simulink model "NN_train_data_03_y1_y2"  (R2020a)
settings: Solver=VariableStepAuto  StartTime=0.0  StopTime=300  RelTol=1e-3
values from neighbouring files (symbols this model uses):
  C = 6.3000e-04    (= 0.00063)    [maglev_init.m]
  g = 9.80    (= 9.8)    [maglev_init.m]
  K = 1.0e+03 * [-2.4567   -0.1235    0.0237]    [maglev_init.m]
  L1 = 0.6000    (= 0.6)    [maglev_init.m]
  m = 0.0300    (= 0.03)    [maglev_init.m]
  mpert = 0    [maglev_init.m]
  R = 45    [maglev_init.m]
  Ts = 0.005    [maglev_init.m]    (also in train_net.m)
  x1_0 = 0.1    [maglev_init.m]
  x1_d = 0.05    [maglev_init.m]
  x2_0 = 0    [maglev_init.m]
  x2_d = 0    [maglev_init.m]
  x3_0 = 0.2    [maglev_init.m]

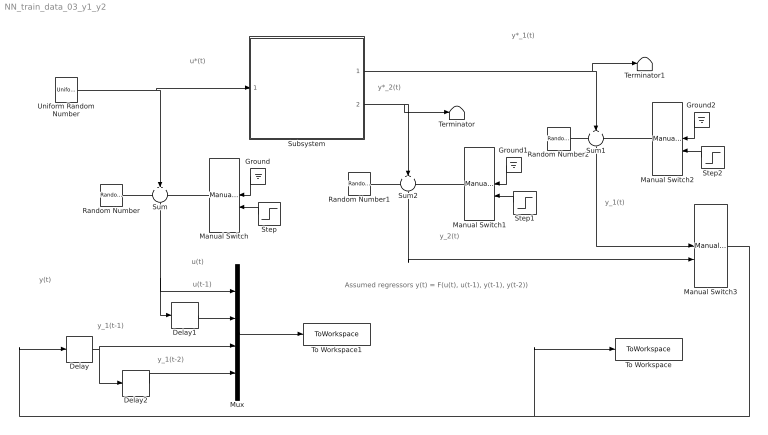
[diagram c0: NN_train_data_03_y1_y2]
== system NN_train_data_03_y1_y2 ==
  note: y(t)
  note: y_1(t-1)
  note: Assumed regressors y(t) = F(u(t), u(t-1), y(t-1), y(t-2))
  note: y_2(t)
  note: y*_1(t)
  note: u(t)
  note: u*(t)
  note: y*_2(t)
  note: y_1(t)
  note: u(t-1)
  note: y_1(t-2)
  Delay : Delay  DelayLength=1  SampleTime=Ts
  Delay1 : Delay  DelayLength=1  SampleTime=Ts
  Delay2 : Delay  DelayLength=1  SampleTime=Ts
  Ground : Ground
  Ground1 : Ground
  Ground2 : Ground
  Manual Switch : ManualSwitch
  Manual Switch1 : ManualSwitch
  Manual Switch2 : ManualSwitch
  Manual Switch3 : ManualSwitch  CurrentSetting=0
  Mux : Mux
  Random Number : RandomNumber  Variance=1e-9  Seed=1  SampleTime=Ts
  Random Number1 : RandomNumber  Variance=1e-6  Seed=3  SampleTime=Ts
  Random Number2 : RandomNumber  Variance=1e-9  Seed=2  SampleTime=Ts
  Step : Step  Time=150  SampleTime=0
  Step1 : Step  Time=150  SampleTime=0
  Step2 : Step  Time=150  SampleTime=0
  Subsystem : Subsystem
  Sum : Sum  Inputs=+++
  Sum1 : Sum  Inputs=+++
  Sum2 : Sum  Inputs=+++
  Terminator : Terminator
  Terminator1 : Terminator
  To Workspace : ToWorkspace  VariableName=Tsim  SampleTime=Ts
  To Workspace1 : ToWorkspace  VariableName=Psim  SampleTime=Ts
  Uniform Random Number : UniformRandomNumber  Minimum=x1_d*0.9  Maximum=x1_d*1.1  Seed=1  SampleTime=0.5
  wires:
  Uniform Random Number/1 -> Subsystem/1(In1), Sum/2
  Subsystem/1(Out1) -> Terminator1/1, Sum1/2
  Subsystem/2(Out2) -> Terminator/1, Sum2/2
  Random Number/1 -> Sum/1
  Manual Switch/1 -> Sum/3
  Manual Switch2/1 -> Sum1/3
  Manual Switch1/1 -> Sum2/3
  Random Number1/1 -> Sum2/1
  Sum/1 -> Delay1/1, Mux/1
  Ground/1 -> Manual Switch/1
  Step/1 -> Manual Switch/2
  Ground1/1 -> Manual Switch1/1
  Step1/1 -> Manual Switch1/2
  Sum2/1 -> Manual Switch3/2
  Random Number2/1 -> Sum1/1
  Ground2/1 -> Manual Switch2/1
  Step2/1 -> Manual Switch2/2
  Delay1/1 -> Mux/2
  Delay/1 -> Delay2/1, Mux/3
  Delay2/1 -> Mux/4
  Mux/1 -> To Workspace1/1
  Sum1/1 -> Manual Switch3/1
  Manual Switch3/1 -> To Workspace/1, Delay/1

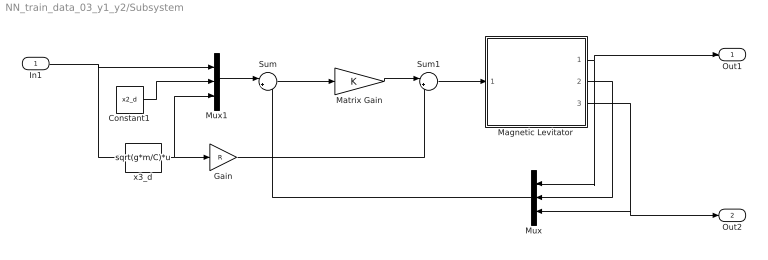
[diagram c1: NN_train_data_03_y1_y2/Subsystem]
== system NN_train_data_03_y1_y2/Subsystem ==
  In1 : Inport
  Constant1 : Constant  Value=x2_d
  Gain : Gain  Gain=R
  Magnetic Levitator : Subsystem  mask{m=m+mpert, R=R, L1=L1, C=C, g=g}
      mask prompts: m "ball's mass (m)"; R "Electromagnet's resistance (R)"; L1 "Electromagnet's inductance (L1)"; C "Magnetic force constant (C)"; g "Gravitational acceleration (g)"
  Matrix Gain : Gain  Gain=K  Multiplication=Matrix(K*u)  SaturateOnIntegerOverflow=on
  Mux : Mux  Inputs=3
  Mux1 : Mux  Inputs=3
  Sum : Sum  Inputs=|+-  InputSameDT=on  SaturateOnIntegerOverflow=on
  Sum1 : Sum  Inputs=|++  InputSameDT=on  SaturateOnIntegerOverflow=on
  x3_d : Fcn  Expr=sqrt(g*m/C)*u
  Out1 : Outport
  Out2 : Outport  Port=2
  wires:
  In1/1 -> x3_d/1, Mux1/1
  Magnetic Levitator/2(x2) -> Mux/2
  x3_d/1 -> Mux1/3, Gain/1
  Mux1/1 -> Sum/1
  Gain/1 -> Sum1/2
  Mux/1 -> Sum/2
  Constant1/1 -> Mux1/2
  Sum/1 -> Matrix Gain/1
  Sum1/1 -> Magnetic Levitator/1(u)
  Magnetic Levitator/1(x1) -> Out1/1, Mux/1
  Magnetic Levitator/3(x3) -> Out2/1, Mux/3
  Matrix Gain/1 -> Sum1/1

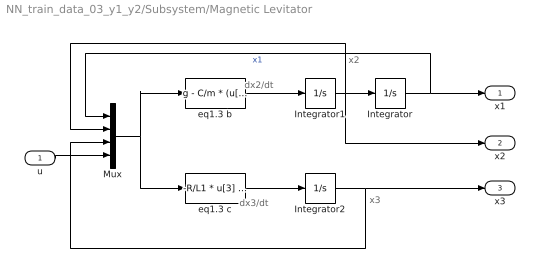
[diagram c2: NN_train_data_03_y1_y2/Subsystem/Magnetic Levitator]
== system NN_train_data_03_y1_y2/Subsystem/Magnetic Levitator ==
  note: x2
  note: x3
  note: dx2/dt
  note: dx3/dt
  u : Inport
  Integrator : Integrator  InitialCondition=x1_0
  Integrator1 : Integrator  InitialCondition=x2_0
  Integrator2 : Integrator  InitialCondition=x3_0
  Mux : Mux
  eq1.3 b : Fcn  Expr=g - C/m * (u[3] / u[1])^2
  eq1.3 c : Fcn  Expr=-R/L1 * u[3] + (2*C)/L1 * ( u[2] * u[3] / u[1]^2 ) + 1/L1 * u[4]
  x1 : Outport
  x2 : Outport  Port=2
  x3 : Outport  Port=3
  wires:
  eq1.3 b/1 -> Integrator1/1
  Integrator1/1 -> Integrator/1, Mux/2, x2/1
  eq1.3 c/1 -> Integrator2/1
  Mux/1 -> eq1.3 b/1, eq1.3 c/1
  Integrator/1 -> Mux/1, x1/1  "x1"
  Integrator2/1 -> Mux/3, x3/1
  u/1 -> Mux/4
